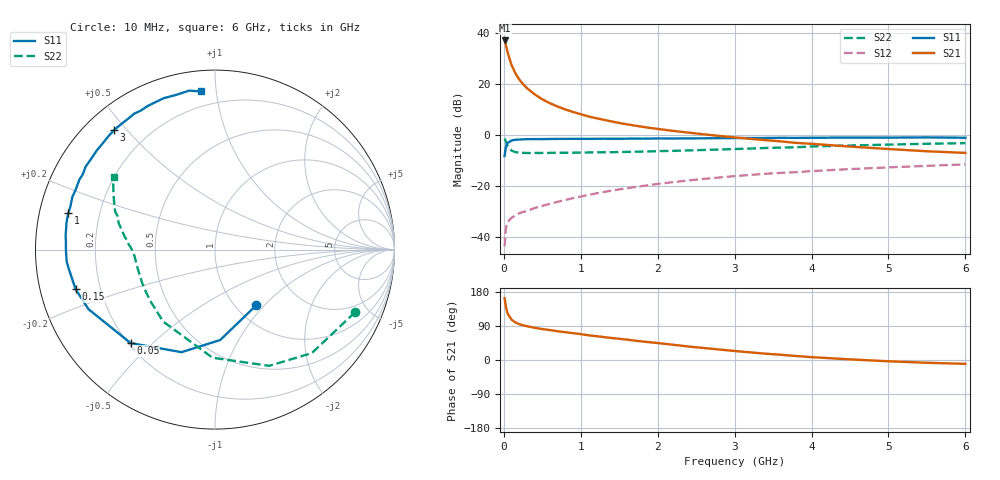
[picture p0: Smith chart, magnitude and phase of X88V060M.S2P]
! SIEMENS Small Signal Semiconductors
! BFP136W
! Si NPN RF Bipolar Junction Transistor in SOT343
! VCE = 8 V  IC = 60 mA
! Common Emitter S-Parameters:  September  1994
# GHz  S  MA  R  50
!  f  S11  S21  S12  S22
! GHz  MAG  ANG  MAG  ANG  MAG  ANG  MAG  ANG
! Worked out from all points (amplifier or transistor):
!   40 points, 10 MHz to 6 GHz, reference 50 ohm
!   highest |S21| = 37.2 dB at 10 MHz (marker M1)
!   |S21| within 3 dB of that: start of sweep to 36.21 MHz
!   unconditionally stable (mu >= 1): 764.4 MHz to 2.954 GHz
!   at 200 MHz: K = 0.55, MSG = 26.3 dB, |S12| = -30.8 dB
!   at 1.5 GHz: K = 1.11, MAG = 11.1 dB, |S12| = -21.4 dB
!   at 6 GHz: K = 0.96, MSG = 2.3 dB, |S12| = -11.6 dB
!   S11 on the Smith chart (normalised r, x): 10 MHz: 1.23, -0.90; 50 MHz: 0.21, -0.43; 150 MHz: 0.11, -0.14; 1 GHz: 0.09, +0.12; 3 GHz: 0.08, +0.46; 6 GHz: 0.11, +0.91
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0.01  0.3862 -53.6  72.58 163.0  0.0065 72.4  0.8547 -24.1
0.02  0.5046 -86.7  64.32 148.3  0.0116 60.3  0.7897 -46.9
0.03  0.6014 -108.1  56.33 137.2  0.0152 52.9  0.7145 -65.0
0.05  0.7015 -132.1  41.88 122.4  0.0195 41.8  0.6026 -91.3
0.1  0.7793 -154.8  23.9 106.3  0.0235 34.4  0.4941 -125.8
0.15  0.8072 -164.1  16.42 99.1  0.0261 34.6  0.4603 -141.6
0.2  0.8137 -169.1  12.39 94.7  0.0289 35.5  0.4501 -150.4
0.25  0.8223 -172.8  10.02 91.6  0.0305 37.1  0.446 -156.1
0.3  0.8292 -175.5  8.379 89.2  0.0321 38.6  0.4428 -159.8
0.4  0.8305 -179.8  6.323 85.1  0.0365 41.7  0.4431 -165.1
0.5  0.8319 177.0  5.044 81.7  0.0403 44.6  0.4436 -168.4
0.6  0.8361 174.5  4.214 79.0  0.0444 46.6  0.4452 -170.7
0.8  0.8407 170.0  3.179 73.3  0.0529 50.5  0.4479 -173.6
1  0.8419 166.0  2.564 68.4  0.0616 52.6  0.451 -175.9
1.1  0.8408 163.3  2.322 65.2  0.0663 53.2  0.4538 -176.7
1.5  0.8455 156.4  1.727 56.0  0.0851 54.6  0.4623 -179.8
2.2  0.8554 143.9  1.206 40.2  0.1182 52.0  0.4878 175.1
3  0.8717 130.1  0.899 23.8  0.1553 46.3  0.5301 168.6
3.2  0.8729 126.9  0.842 20.2  0.1638 44.6  0.5413 166.6
4.5  0.8907 108.7  0.592 1.7  0.2135 34.1  0.622 154.7
5.5  0.8974 99.2  0.479 -7.3  0.2474 26.0  0.6729 147.4
6  0.8843 95.0  0.445 -10.1  0.2642 21.8  0.6914 144.3
